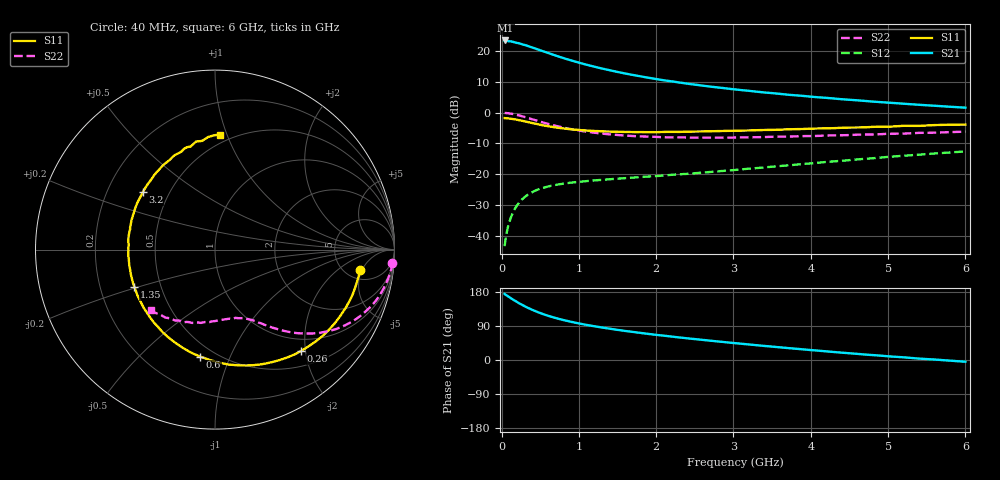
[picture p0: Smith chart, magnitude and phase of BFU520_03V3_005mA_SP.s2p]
! Filename:  P:\Prog\Test\Noise\ATS_data\Testdata_Net\03 Spar\BFU520_APG2013_37_A05_03p3V_005mA_SP_CM01_D.s2p
! Date/Time: Fri 26/Apr/2013 13:00:02
! BFU520_APG2013_37_A05_03p3V_1to20mA_SP_CM01_Bias4_R.s2p
! MDIF S-parameter v. bias file
! BFU520_APG2013_37_A05_03p3V_1to20mA_SP_CM01
! Date/time Tue Apr 23 14:11:50 2013
! VAR V_out= 3.3000
! VAR I_out= 4.9950
! VAR V_in= 0.8302
! VAR I_in= 0.0575
! Device data file deembeded for feedlines and parallel
! Original file: \03 Spar\BFU520_APG2013_37_A05_03p3V_005mA_SP_CM01_R.s2p
! Feed-files: PR047V01_250413_Feed1.s2p, PR047V01_250413_Feed2.s2p
! Parallel-file: PR047V01_250413_Par.s2p
# MHz S MA R 50
!  Freq-MHz  S11-mag  S11-arg  S21-mag  S21-arg  S12-mag  S12-arg  S22-mag  S22-arg
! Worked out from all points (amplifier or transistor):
!   98 points, 40 MHz to 6 GHz, reference 50 ohm
!   highest |S21| = 23.5 dB at 50 MHz (marker M1)
!   |S21| within 3 dB of that: start of sweep to 478 MHz
!   unconditionally stable (mu >= 1): 2.276 GHz to 4.517 GHz
!   at 300 MHz: K = 0.19, MSG = 24.7 dB, |S12| = -27.5 dB
!   at 1.6 GHz: K = 0.82, MSG = 17.0 dB, |S12| = -21.3 dB
!   at 6 GHz: K = 0.86, MSG = 7.1 dB, |S12| = -12.6 dB
!   S11 on the Smith chart (normalised r, x): 40 MHz: 6.69, -4.60; 260 MHz: 0.77, -1.92; 600 MHz: 0.42, -0.78; 1.35 GHz: 0.35, -0.19; 3.2 GHz: 0.36, +0.31; 6 GHz: 0.43, +0.95
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40  0.8166 -8.1  14.96 174.3  0.006719 85.3  0.9911 -4.2
50  0.8146 -10.1  14.99 172.3  0.008309 84.4  0.9895 -5.3
70  0.8103 -13.9  14.76 170.2  0.01163 82.5  0.9842 -7.6
140  0.79 -27.7  14.31 160.6  0.02251 75.3  0.9553 -14.9
220  0.7588 -42.5  13.56 150.8  0.03339 68.0  0.9066 -22.4
260  0.7413 -49.6  13.09 146.2  0.03817 64.7  0.8799 -25.8
320  0.713 -59.7  12.45 139.8  0.04438 60.2  0.8368 -30.4
400  0.6777 -71.9  11.49 132.2  0.05111 55.4  0.7793 -35.5
500  0.637 -85.6  10.38 124.0  0.05789 50.5  0.7154 -40.8
600  0.6022 -97.8  9.413 116.8  0.06287 46.7  0.6588 -45.0
700  0.5755 -108.3  8.517 110.8  0.06673 44.0  0.6118 -48.4
800  0.5544 -117.7  7.753 105.5  0.06999 41.9  0.5724 -51.2
1050  0.5169 -137.3  6.277 94.5  0.07594 38.9  0.5012 -56.7
1350  0.4949 -155.2  5.064 84.2  0.08163 37.7  0.4499 -61.5
1600  0.4853 -167.6  4.343 76.7  0.08601 37.7  0.4247 -65.3
2050  0.4843 175.2  3.445 65.3  0.09385 38.9  0.4009 -72.0
2450  0.4918 161.6  2.912 56.2  0.102 40.3  0.3926 -78.3
3100  0.5107 143.4  2.333 43.0  0.1193 42.6  0.3957 -88.2
3200  0.5137 141.5  2.271 41.0  0.1229 42.8  0.3977 -89.5
4100  0.5538 120.6  1.779 24.6  0.1533 42.6  0.4191 -104.5
5200  0.6113 99.9  1.4 7.1  0.199 38.7  0.4562 -122.9
6000  0.6416 87.4  1.208 -4.6  0.2344 33.6  0.4913 -136.3
